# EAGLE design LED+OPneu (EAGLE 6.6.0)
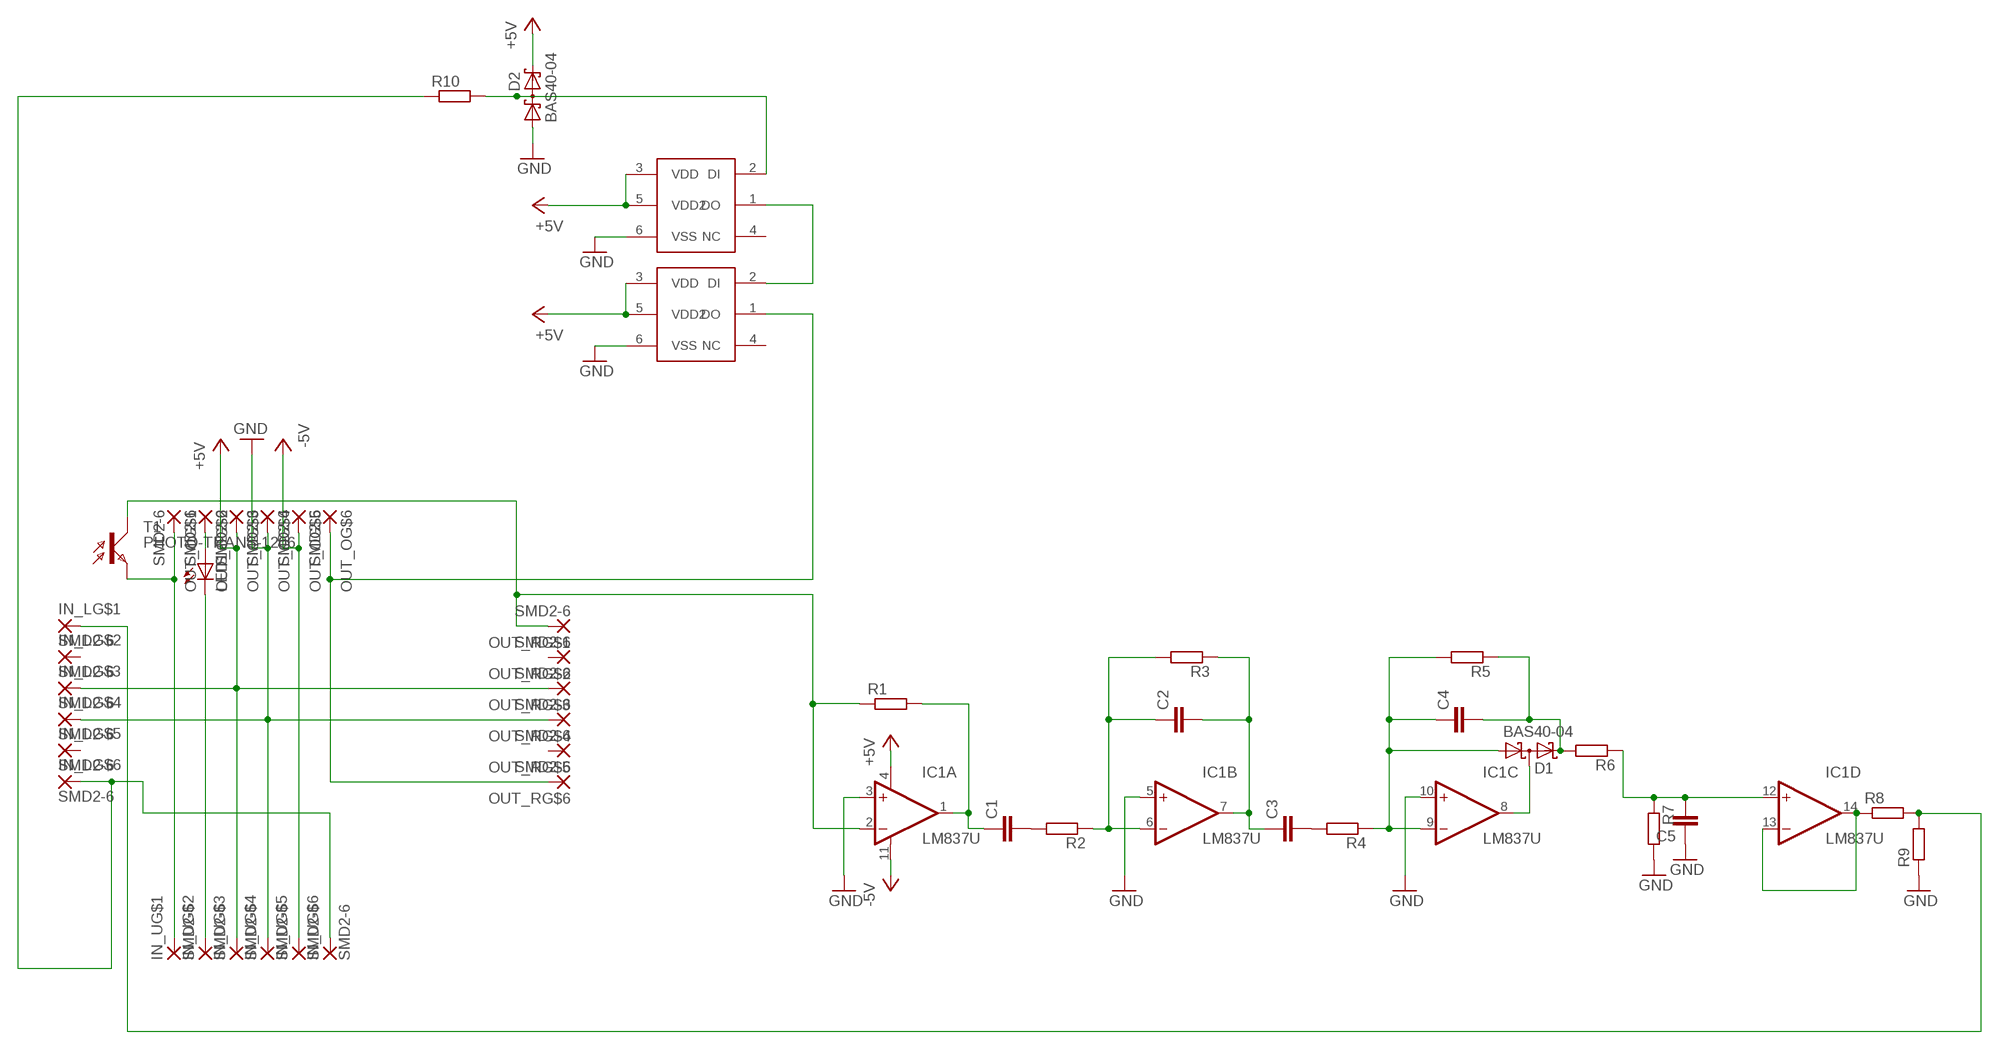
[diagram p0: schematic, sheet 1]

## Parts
C1  C-EUC1206  [C1206]
C2  C-EUC1206  [C1206]
C3  C-EUC1206  [C1206]
C4  C-EUC1206  [C1206]
C5  C-EUC1206  [C1206]
D1  BAS40-04  [SOT23]
D2  BAS40-04  [SOT23]
IC1  LM837U  [SO14]
IN_L  SMD2-6  [SMD1,27-2,54-6]
IN_U  SMD2-6  [SMD1,27-2,54-6]
LED1  LED3MM  [LED3MM]
OUT_O  SMD2-6  [SMD1,27-2,54-6]
OUT_R  SMD2-6  [SMD1,27-2,54-6]
R1  R-EU_M1206  [M1206]
R2  R-EU_M1206  [M1206]
R3  R-EU_M1206  [M1206]
R4  R-EU_M1206  [M1206]
R5  R-EU_M1206  [M1206]
R6  R-EU_M1206  [M1206]
R7  R-EU_M1206  [M1206]
R8  R-EU_M1206  [M1206]
R9  R-EU_M1206  [M1206]
R10  R-EU_M1206  [M1206]
T1  PHOTO-TRANS-1206  [1206]
U$1  LED_SMD5050  [CLN6A]
U$2  LED_SMD5050  [CLN6A]

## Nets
+5V: D2.2(C2) IC1.4(A:V+) IN_L.3 IN_U.3 OUT_O.3 OUT_R.3 U$1.3(VDD) U$1.5(VDD2) U$2.3(VDD) U$2.5(VDD2)
-5V: IC1.11(A:V-) IN_U.5 OUT_O.5
GND: C5.1 D2.1(A1) IC1.3(A:+IN) IC1.5(B:+IN) IC1.10(C:+IN) IN_L.4 IN_U.4 OUT_O.4 OUT_R.4 R7.2 R9.1 U$1.6(VSS) U$2.6(VSS)
N$1: IC1.2(A:-IN) OUT_R.1 R1.1 T1.A(C)
N$2: C1.1 IC1.1(A:OUT) R1.2
N$3: C1.2 R2.2
N$4: IN_U.1 OUT_O.1 T1.C(E)
N$5: D1.3(C1A2) IC1.8(C:OUT)
N$6: U$1.1(DO) U$2.2(DI)
N$7: D2.3(C1A2) R10.2 U$1.2(DI)
N$8: IC1.13(D:-IN) IC1.14(D:OUT) R8.1
N$9: C2.1 IC1.6(B:-IN) R2.1 R3.2
N$10: C2.2 C3.1 IC1.7(B:OUT) R3.1
N$11: C4.2 D1.2(C2) R5.1 R6.2
N$13: LED1.A OUT_O.2
N$14: C3.2 R4.2
N$15: C4.1 D1.1(A1) IC1.9(C:-IN) R4.1 R5.2
N$17: IN_L.6 IN_U.6 R10.1
N$18: IN_L.1 R8.2 R9.2
N$19: C5.2 IC1.12(D:+IN) R6.1 R7.1
N$21: OUT_O.6 OUT_R.6 U$2.1(DO)
N$25: IN_U.2 LED1.K(C)
Unconnected: IN_L.2 IN_L.5 OUT_R.2 OUT_R.5 U$1.4(NC) U$2.4(NC)

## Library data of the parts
C1-C5 = resistor:C-EU: CAPACITOR, European symbol
D1 D2 = diode:BAS40-04: Silicon Schottky Diodes General-purpose diode for high-speed switching
IC1 = #mylib:LM837: Operational Amplifiers; OC_FARNELL: unknown; OC_NEWARK: unknown
IN_L IN_U OUT_O OUT_R = #mylib:SMD2-6
LED1 = led:LED: LED
R1-R10 = resistor:R-EU_: RESISTOR, European symbol
T1 = #mylib:PHOTO-TRANS-1206: PHOTO TRANSISTOR
U$1 U$2 = #mylib:LED_SMD5050

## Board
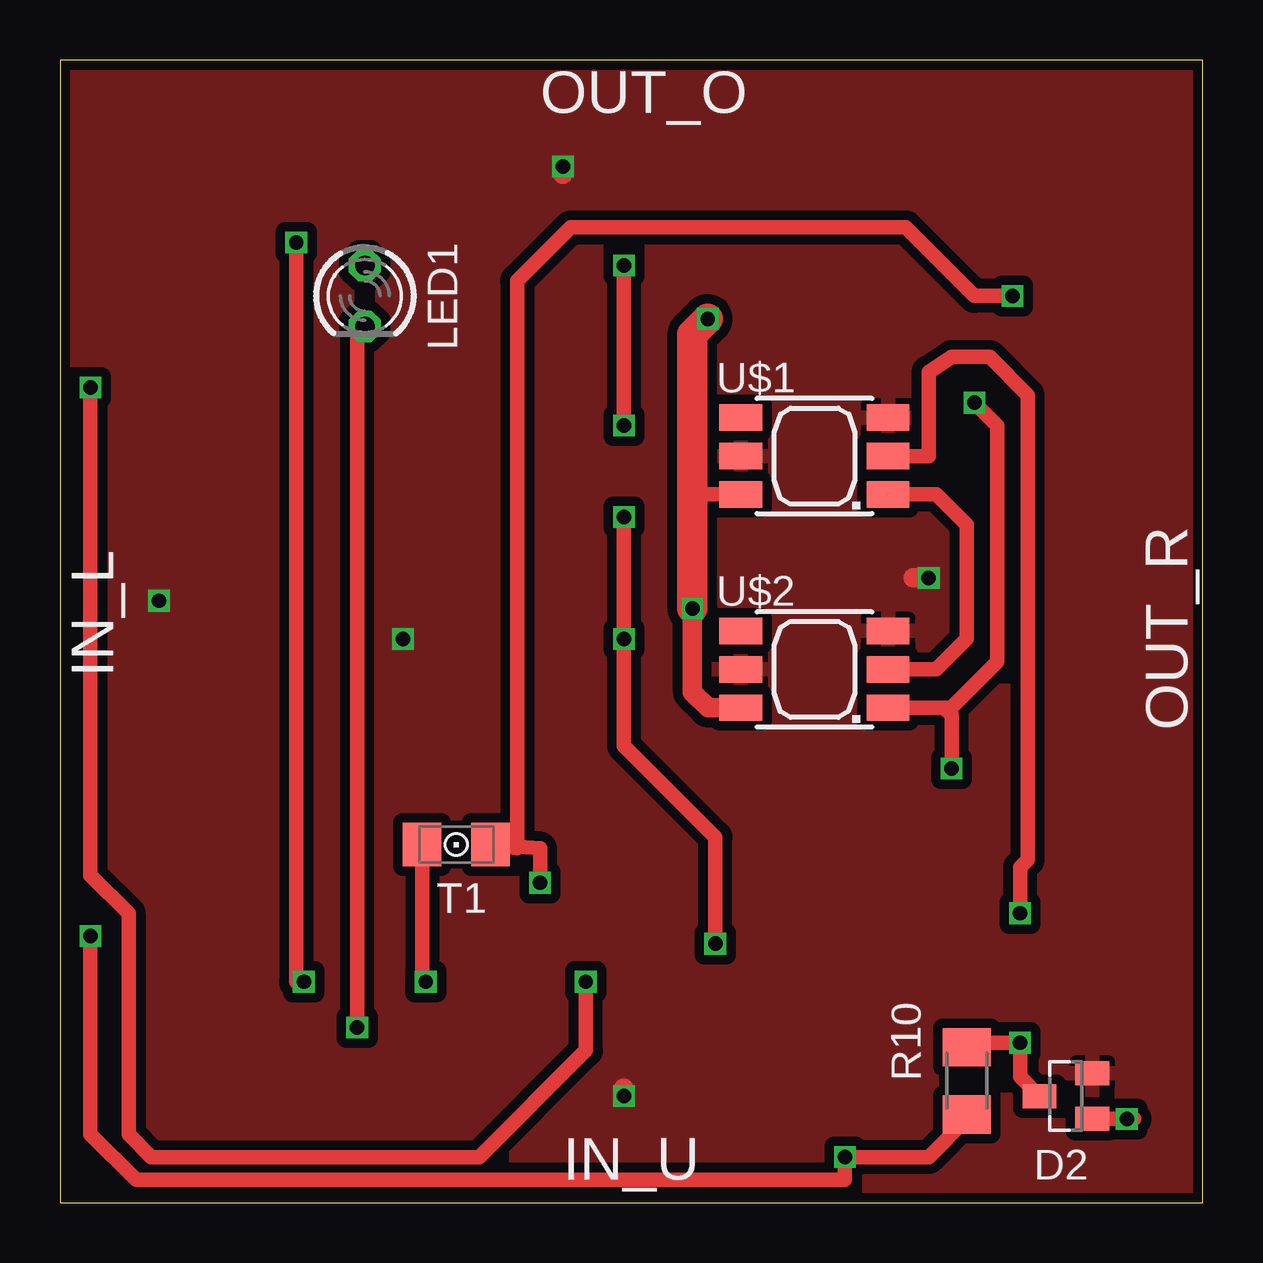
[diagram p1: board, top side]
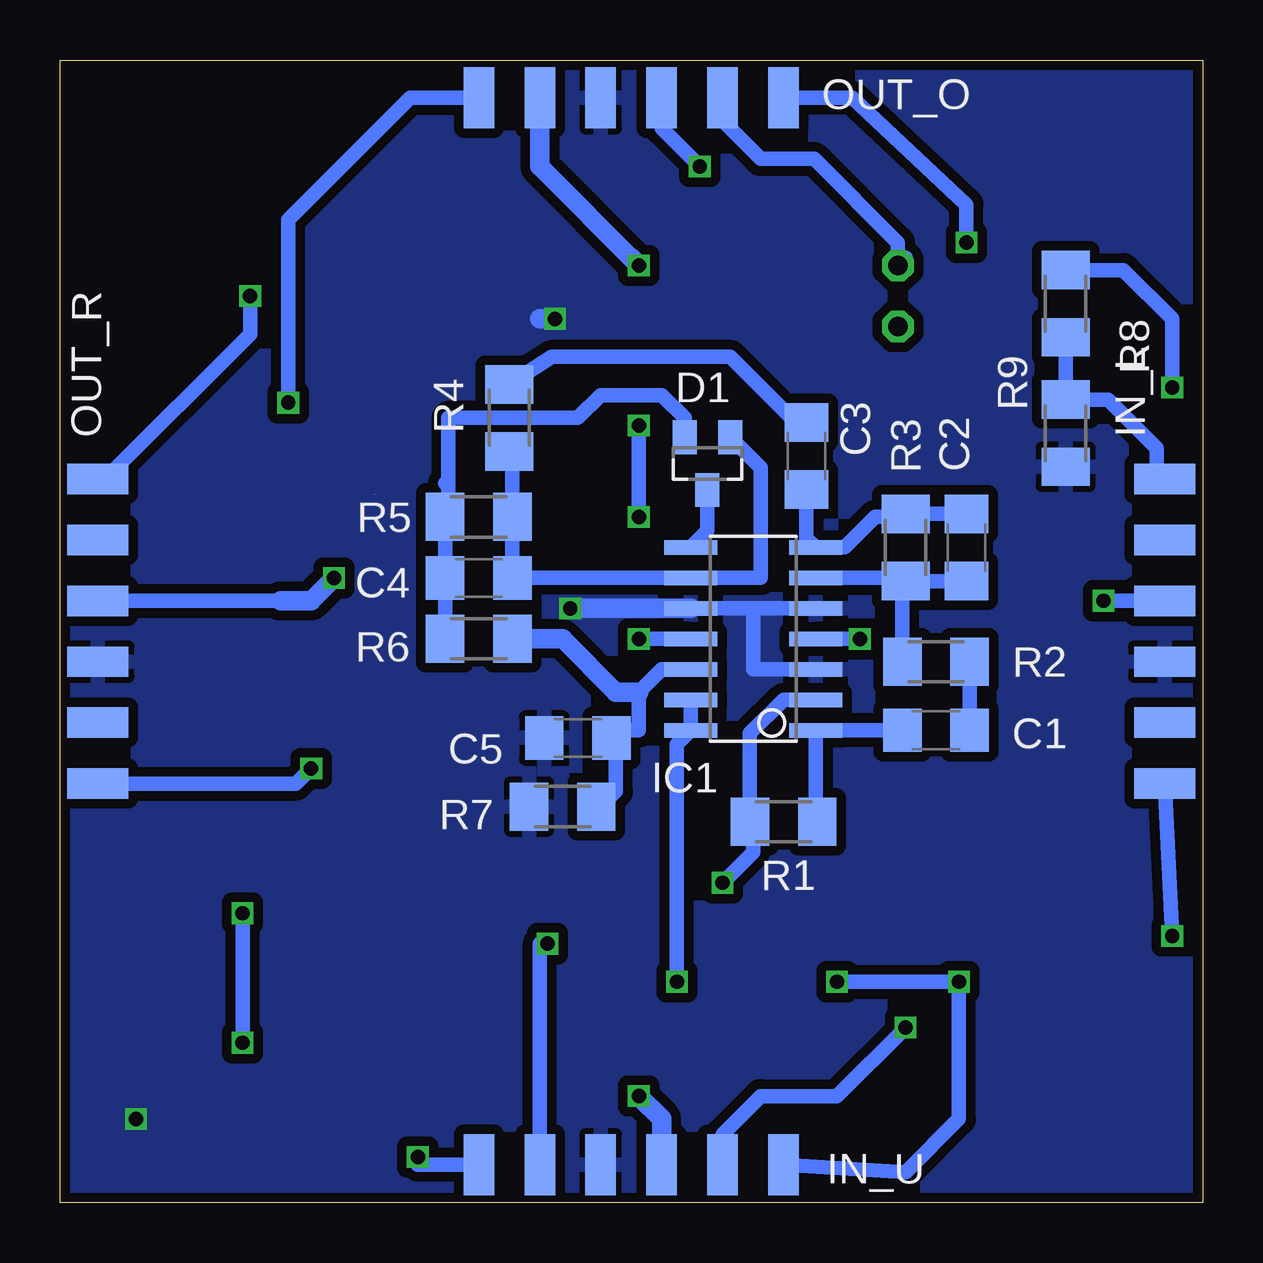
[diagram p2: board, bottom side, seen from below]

Size 47.61 x 47.62 mm. Coordinates in mm from the lower left corner, seen from the top.
Outline: 0,0 47.61,0 47.61,47.62 0,47.62 0,0
Copper layers (1*16): Top 0.035mm / dielectric 1.5mm / Bottom 0.035mm
Design rules "Elecrow_2-layer_eagle_rule": minimum track width 6mil, minimum drill 12mil, track to track 6mil, track to pad 6mil, pad to pad 6mil, via to via 6mil, smd to smd 0mil, copper to edge 10mil, drill to drill 10mil, minimum pad ring 10mil, minimum via ring 6mil, stop-mask expansion 2mil, vias tented up to drill 100mil, thermal gap 10mil

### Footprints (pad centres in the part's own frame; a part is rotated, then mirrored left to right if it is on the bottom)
C1206 = smd 1.6 x 1.8: 1 -1.4,0; 2 1.4,0
SOT23 = smd 1 x 1.4: 1 -0.95,-1.1; 2 0.95,-1.1; 3 0,1.1
SO14 = smd 0.61 x 2.21: 1 -3.81,-2.603; 2 -2.54,-2.603; 3 -1.27,-2.603; 4 0,-2.603; 5 1.27,-2.603; 6 2.54,-2.603; 7 3.81,-2.603; 8 3.81,2.603; 9 2.54,2.603; 10 1.27,2.603; 11 0,2.603; 12 -1.27,2.603; 13 -2.54,2.603; 14 -3.81,2.603
SMD1,27-2,54-6 = smd 1.27 x 2.54: 1 0,0; 2 2.54,0; 3 5.08,0; 4 7.62,0; 5 10.16,0; 6 12.7,0
LED3MM = drill 0.813 octagon: A -1.27,0; K 1.27,0
M1206 = smd 1.6 x 2: 1 -1.4,0; 2 1.4,0
1206 = smd 1.6 x 1.803: A -1.422,0; C 1.422,0
CLN6A = smd 1.778 x 1.1: 1 3.071,-1.6; 2 3.071,0; 3 3.071,1.6; 4 -3.071,1.6; 5 -3.071,0; 6 -3.071,-1.6

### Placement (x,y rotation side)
C1  11.11,19.68 0 bottom
C2  9.84,27.3 90 bottom
C3  16.51,31.11 90 bottom
C4  30.16,26.04 180 bottom
C5  26.04,19.37 0 bottom
D1  20.64,30.8 180 bottom
D2  41.91,4.45 90 top
IC1  18.73,23.5 90 bottom
IN_L  1.59,30.16 270 bottom
IN_U  17.46,1.59 180 bottom
LED1  12.7,37.78 270 top
OUT_O  17.46,46.04 180 bottom
OUT_R  46.04,30.16 270 bottom
R1  17.46,15.88 0 bottom
R2  11.11,22.54 0 bottom
R3  12.38,27.3 270 bottom
R4  28.89,32.7 90 bottom
R5  30.16,28.57 0 bottom
R6  30.16,23.5 180 bottom
R7  26.67,16.51 180 bottom
R8  5.71,37.47 270 bottom
R9  5.71,32.07 90 bottom
R10  37.78,5.08 90 top
T1  16.51,14.92 180 top
U$1  31.43,31.11 0 top
U$2  31.43,22.23 0 top

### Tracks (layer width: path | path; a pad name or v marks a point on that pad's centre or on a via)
+5V  (via drill 0.6)
  Top 0.813: v20.95,43.18 20.95,42.86 | v36.2,26.04 35.56,26.04 | v23.5,4.45 23.5,4.76
  Bottom 0.61: IN_L.3 v4.13,25.08 | OUT_R.3 38.42,25.08 | v14.29,23.5 IC1.4 | OUT_O.3 22.54,44.77 v20.95,43.18
  Bottom 0.813: 38.42,25.08 37.15,25.08 v36.2,26.04 | IN_U.3 22.54,3.49 v23.5,4.45
  pour Top (isolate 0.406): 0.32,47.31 47.31,47.31 47.31,0.32 0.32,0.32
-5V  (via drill 0.6)
  Top 0.61: v27.3,10.79 27.3,15.24 23.5,19.05 v23.5,23.5 v23.5,28.57 | v23.5,39.05 v23.5,32.38
  Bottom 0.61: IC1.11 v23.5,23.5 | v23.5,32.38 v23.5,28.57 | IN_U.5 27.62,10.79 v27.3,10.79
  Bottom 0.813: 23.81,39.37 v23.5,39.05 27.62,43.18 OUT_O.5
GND  (via drill 0.6)
  Top 0.61: D2.1 44.77,3.5 v44.45,3.49 | U$1.6 26.36,29.52
  Top 0.813: U$2.6 27,20.62 26.35,21.27 v26.35,24.77 | 26.36,29.52 26.35,29.53
  Top 1.27: v26.35,24.77 26.35,29.53 26.35,36.2 v26.99,36.83
  Bottom 0.61: IC1.10 18.73,24.77 | 18.73,24.77 IC1.5 | IC1.3 18.73,22.23 18.73,24.77
  Bottom 0.813: v26.99,36.83 27.62,36.83 | IC1.10 v26.35,24.77
  pour Bottom (isolate 0.406): 0.32,47.31 47.31,47.31 47.31,0.32 0.32,0.32
N$1  (via drill 0.6)
  Top 0.61: v20,13.34 20,14.77 T1.A 19.05,14.77 19.05,38.42 21.27,40.64 35.24,40.64 38.1,37.78 v39.69,37.78
  Bottom 0.61: IC1.2 17.46,20.95 18.86,19.55 R1.1 18.73,15.88 18.73,14.61 v20,13.34 | OUT_R.1 45.72,30.16 39.69,36.2 v39.69,37.78
N$2
  Bottom 0.61: C1.1 IC1.1 16.13,15.94 R1.2
N$3
  Bottom 0.61: C1.2 R2.2
N$4  (via drill 0.6)
  Top 0.61: v9.84,40.01 9.84,9.21 v10.16,9.21 | T1.C 15.09,9.36 v15.24,9.21
  Bottom 0.61: v15.24,9.21 v10.16,9.21 10.16,3.49 12.38,1.27 IN_U.1 | v9.84,40.01 9.84,41.59 14.61,46.04 OUT_O.1
N$5
  Bottom 0.61: 21.27,27.37 IC1.8 20.64,28 D1.3
N$6  (1 unrouted)
  Top 0.61: U$2.2 36.51,22.23 37.78,23.5 37.78,28.26 36.51,29.53 34.52,29.53
N$7  (via drill 0.6)
  Top 0.61: 40.96,4.3 D2.3 40.01,5.25 v40.01,6.67 37.97,6.67 R10.2 | v40.01,12.06 40.01,13.97 40.32,14.29 40.32,33.66 38.73,35.24 37.15,35.24 36.2,34.61 36.2,31.11 U$1.2
  Bottom 0.61: v40.01,6.67 v40.01,12.06
N$8  (via drill 0.6)
  Top 0.61: v1.27,33.97 1.27,13.65 2.86,12.06 2.86,2.86 3.81,1.91 17.46,1.91 21.91,6.35 v21.91,9.21
  Bottom 0.61: IC1.13 IC1.14 21.91,19.11 v21.91,9.21 | R8.1 3.31,38.87 1.27,36.83 v1.27,33.97
N$9
  Bottom 0.61: IC1.6 12.51,26.04 R3.2 | R3.2 C2.1 | R2.1 12.51,25.77 R3.2
N$10
  Bottom 0.61: C2.2 R3.1 12.51,28.57 13.65,28.57 14.92,27.3 IC1.7 16.51,27.69 C3.1
N$11
  Bottom 0.61: 31.69,26.16 C4.2 | C4.2 R5.1 31.43,28.7 31.43,29.84 | 31.43,29.84 31.43,32.7 26.04,32.7 25.08,33.66 22.54,33.66 21.59,32.7 D1.2 | 31.56,29.98 31.43,29.84 | C4.2 R6.2
N$13
  Bottom 0.61: 12.38,39.37 LED1.A 12.7,40.01 16.19,43.5 18.41,43.5 20,45.09 OUT_O.2
N$14
  Bottom 0.61: R4.2 27.12,35.24 19.68,35.24 16.96,32.52 C3.2
N$15
  Bottom 0.61: R4.1 28.76,30.86 R5.2 C4.1 IC1.9 18.41,26.04 18.41,30.62 D1.1
N$17  (via drill 0.6)
  Top 0.61: R10.1 37.78,3.49 36.2,1.91 v32.7,1.91 32.7,0.95 3.17,0.95 1.27,2.86 v1.27,11.11
  Bottom 0.61: v1.27,11.11 IN_L.6 | IN_U.6 32.7,1.59 v32.7,1.91
N$18
  Bottom 0.61: R8.2 R9.2 3.94,33.47 1.91,31.43 1.91,30.48 IN_L.1
N$19
  Bottom 0.61: IC1.12 22.54,22.23 23.5,21.27 23.5,19.68 24.32,19.68 C5.2 | 24.45,19.55 C5.2 | 25.27,16.7 R7.1 25.08,16.51 24.45,17.14 24.45,19.18 C5.2
  Bottom 0.813: 23.5,21.27 24.45,21.27 26.67,23.5 R6.1
N$21  (via drill 0.6)
  Top 0.61: U$2.1 36.83,20.62 | 36.83,20.62 37.13,20.62 39.05,22.54 39.05,32.38 v38.1,33.34 | v37.15,18.1 37.15,20.31 36.83,20.62
  Bottom 0.61: v38.1,33.34 38.1,40.96 33.02,46.04 OUT_O.6 | OUT_R.6 37.78,17.46 v37.15,18.1
N$25  (via drill 0.6)
  Top 0.61: v12.38,7.3 12.38,36.2 LED1.K
  Bottom 0.61: IN_U.2 20,2.86 18.41,4.45 15.24,4.45 v12.38,7.3

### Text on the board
tNames: OUT_O | IN_L | OUT_R | IN_U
